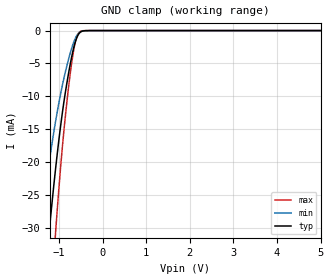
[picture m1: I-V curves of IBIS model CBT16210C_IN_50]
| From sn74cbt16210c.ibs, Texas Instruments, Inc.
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[Model]   CBT16210C_IN_50
Model_type  Input
Vinl=0.8
Vinh=2.0
| variable   typ   min   max
C_comp   4.52pF   2.54pF   8.14pF
[Temperature Range]   40   100   -40
| Ambient temperature   25   85   -40
[Voltage range]   5   4.5   5.5
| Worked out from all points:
|   GND clamp passes 1 mA (typ) near -0.59 V on its own axis
[GND Clamp]
| CBT16210C_IN
|   Voltage   I(typ)   I(min)   I(max)
-5V       -417.7mA   -314mA     -530.4mA
-1.45V    -47.62mA   -31.29mA   -69.62mA
-1.425V   -45.62mA   -29.95mA   -66.79mA
-1.215V   -29.94mA   -19.59mA   -44.09mA
-1.075V   -20.84mA   -13.7mA    -30.44mA
-995mV    -16.23mA   -10.74mA   -23.41mA
-910mV    -11.91mA   -7.942mA   -16.81mA
-750mV    -5.384mA   -3.616mA   -6.969mA
-680mV    -3.115mA   -2.099mA   -3.645mA
-615mV    -1.514mA   -1.041mA   -1.461mA
-495mV    -172.7uA   -149.6uA   -80.07uA
5V        220pA      718pA      41.32pA
